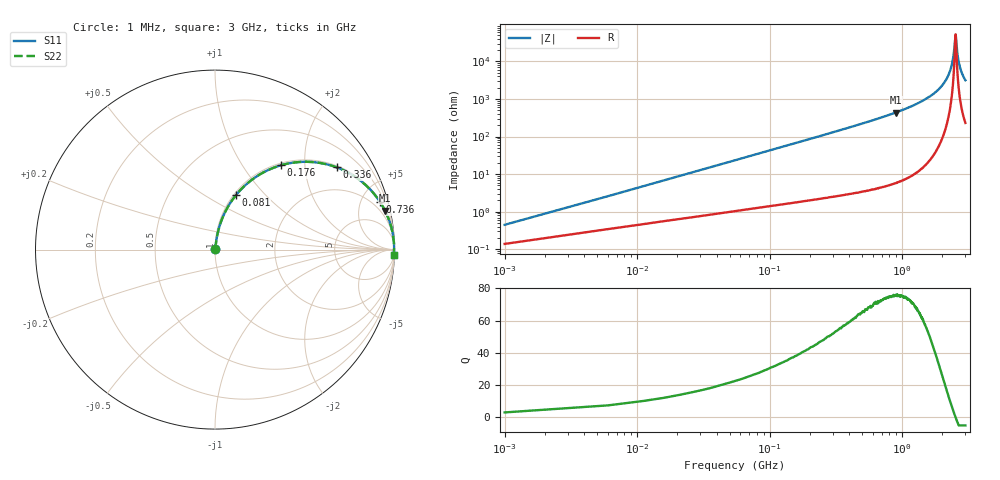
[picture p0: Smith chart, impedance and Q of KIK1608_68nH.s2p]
!version-2
!date-01.2022
!Series
# MHz S RI R 50
!Freq ReS11 ImS11 ReS21 ImS21 ReS12 ImS12 ReS22 ImS22
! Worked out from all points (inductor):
!   601 points, 1 MHz to 3 GHz, reference 50 ohm
!   read as one part in series: L = 68 nH near 16 MHz
!   highest Q = 75.7 at 891 MHz (marker M1), where L = 77.6 nH
!   self-resonance near 2.53 GHz
!   S11 on the Smith chart (normalised r, x): 1 MHz: 1.00, +0.01; 81 MHz: 1.03, +0.69; 176 MHz: 1.04, +1.51; 336 MHz: 1.05, +2.92; 736 MHz: 1.09, +6.87; 3 GHz: 6, -63
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1  0.00142 0.00426  0.9986 -0.00426  0.9986 -0.00426  0.00142 0.00426
21  0.0142 0.0879  0.9858 -0.0879  0.9858 -0.0879  0.0142 0.0879
26  0.019 0.1082  0.981 -0.1082  0.981 -0.1082  0.019 0.1082
46  0.0456 0.1859  0.9544 -0.1859  0.9544 -0.1859  0.0456 0.1859
81  0.116 0.3024  0.884 -0.3024  0.884 -0.3024  0.116 0.3024
176  0.3668 0.4697  0.6332 -0.4697  0.6332 -0.4697  0.3668 0.4697
336  0.6781 0.4582  0.3219 -0.4582  0.3219 -0.4582  0.6781 0.4582
501  0.8286 0.3693  0.1714 -0.3693  0.1714 -0.3693  0.8286 0.3693
736  0.9188 0.2664  0.0812 -0.2664  0.0812 -0.2664  0.9188 0.2664
891  0.9471 0.2173  0.0529 -0.2173  0.0529 -0.2173  0.9471 0.2173
1005  0.9607 0.1877  0.0393 -0.1877  0.0393 -0.1877  0.9607 0.1877
1505  0.9883 0.099  0.0117 -0.099  0.0117 -0.099  0.9883 0.099
2005  0.9965 0.0432  0.00354 -0.0432  0.00354 -0.0432  0.9965 0.0432
2205  0.9976 0.0254  0.00238 -0.0254  0.00238 -0.0254  0.9976 0.0254
2345  0.998 0.014  0.002 -0.014  0.002 -0.014  0.998 0.014
2440  0.9981 0.00667  0.0019 -0.00667  0.0019 -0.00667  0.9981 0.00667
2505  0.9981 0.00183  0.0019 -0.00183  0.0019 -0.00183  0.9981 0.00183
2525  0.9981 0.000364  0.00191 -0.000364  0.00191 -0.000364  0.9981 0.000364
2540  0.9981 -0.000726  0.00192 0.000726  0.00192 0.000726  0.9981 -0.000726
2620  0.998 -0.00644  0.00202 0.00644  0.00202 0.00644  0.998 -0.00644
2720  0.9978 -0.0133  0.00223 0.0133  0.00223 0.0133  0.9978 -0.0133
3000  0.9967 -0.0314  0.0033 0.0314  0.0033 0.0314  0.9967 -0.0314
